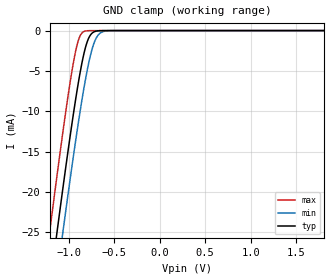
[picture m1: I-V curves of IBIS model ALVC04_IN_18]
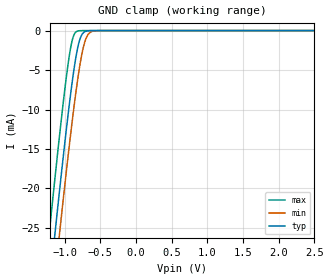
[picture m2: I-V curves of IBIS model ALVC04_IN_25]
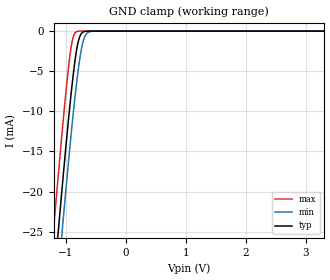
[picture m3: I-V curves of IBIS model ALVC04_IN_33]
| TEXAS INSTRUMENTS INCORPORATED
| Standard Linear and Logic Group
| IBIS Model of SN74ALVC04
| HEX INVERTER
| This file contains package information for the following:
|  SOIC 14-pin (D) package as [Component] ALVC04_D
|  TVSOP 14-pin (DGV) package as [Component] ALVC04_DGV
|  TSSOP 14-pin (PW) package as [Component] ALVC04_PW
| This device can be powered at the following Vccs:
|  1.8 volt Vcc
|  2.5 volt Vcc
|  3.3 volt Vcc
| This file provides unique models under the [Model Selector] for each Vcc.
| For operation at a specific Vcc, select the appropriate model after each
| [Model Selector] keyword.
[IBIS Ver]   3.2
[Comment char]  |_char
[File Name]   sn74alvc04.ibs
[File Rev]   1.1 | x_die
[Date]   March 8, 2002
[Source]   Data created from TI-SPICE simulations at TI-SLL.
[Notes]   The following is an IBIS list for the ALVC04.
   Please contact sllibis@ti.com with questions and
   comments concerning SLL IBIS models.
[Disclaimer] Property of Texas Instruments Incorporated.  Unauthorized
   reproduction and/or distribution is strictly prohibited.
   This product is protected under copyright law.
   Created  2002, (C) Copyright  2002, Texas Instruments
   Incorporated, All Rights Reserved
   UNLESS THERE IS A SIGNED, WRITTEN AGREEMENT TO THE
   CONTRARY, TEXAS INSTRUMENTS (TI) IS PROVIDING THE IBIS
   MODELS  AND WITHOUT ANY WARRANTY, EXPRESSED OR
   IMPLIED.  TI assumes no liability for:
   1) the accuracy of the IBIS models provided to your
   company;
   2) the proper functioning of these IBIS Models in your
   design or for any resulting applications; or
   3) infringement of patents, copyrights or intellectual
   property rights resulting from your use of these IBIS
   models.
   TI provides IBIS Models as a service to our customers.
   You and your company shall not distribute, sell or give
   these models to anyone else without prior written
   permission from TI.
   TI reserves the right to make changes to our products or
   to discontinue any semiconductor product or service
   without notice, and advises our customers to obtain the
   latest version of relevant information to verify, before
   placing orders, that the information being relied on is
   current.
   Please be aware that your receipt and use of the IBIS
   information provided shall serve as acceptance of these
   terms and conditions.  If you do not accept these terms,
   you should return or destroy the IBIS models and any
   other accompanying information immediately.
| Component ALVC04_D 14-pin SOIC
[Component]   ALVC04_D
[Manufacturer]   Texas Instruments, Inc.
[Package]
|   typ   min   max
R_pkg   3.100e-02   2.800e-02   3.400e-02
L_pkg   3.109e-09   2.462e-09   3.889e-09
C_pkg   4.730e-13   3.630e-13   6.280e-13
[Pin]   signal_name   model_name   R_pin   L_pin   C_pin
1   A1   ALVC04_IN   3.300e-02   3.854e-09   6.220e-13
2   Y1   ALVC04_OUT   3.200e-02   3.188e-09   4.730e-13
3   A2   ALVC04_IN   2.800e-02   2.462e-09   3.770e-13
4   Y2   ALVC04_OUT   3.100e-02   2.596e-09   3.630e-13
5   A3   ALVC04_IN   2.800e-02   2.521e-09   3.720e-13
6   Y3   ALVC04_OUT   3.400e-02   3.250e-09   4.760e-13
7   GND   GND   3.400e-02   3.889e-09   6.280e-13
8   Y4   ALVC04_OUT   3.400e-02   3.889e-09   6.280e-13
9   A4   ALVC04_IN   3.400e-02   3.250e-09   4.760e-13
10   Y5   ALVC04_OUT   2.800e-02   2.521e-09   3.720e-13
11   A5   ALVC04_IN   3.100e-02   2.596e-09   3.640e-13
12   Y6   ALVC04_OUT   2.800e-02   2.462e-09   3.770e-13
13   A6   ALVC04_IN   3.200e-02   3.188e-09   4.730e-13
14   VCC   POWER   3.300e-02   3.854e-09   6.220e-13
| Component ALVC04_DGV 14-pin TVSOP
[Component]   ALVC04_DGV
[Manufacturer]   Texas Instruments, Inc.
[Package]
|   typ   min   max
R_pkg   3.500e-02   2.000e-02   4.500e-02
L_pkg   2.499e-09   2.077e-09   2.966e-09
C_pkg   3.610e-13   3.050e-13   4.160e-13
[Pin]   signal_name   model_name   R_pin   L_pin   C_pin
1   A1   ALVC04_IN   2.700e-02   2.717e-09   3.730e-13
2   Y1   ALVC04_OUT   3.700e-02   2.434e-09   3.980e-13
3   A2   ALVC04_IN   3.400e-02   2.200e-09   3.160e-13
4   Y2   ALVC04_OUT   2.000e-02   2.077e-09   3.090e-13
5   A3   ALVC04_IN   3.000e-02   2.147e-09   3.050e-13
6   Y3   ALVC04_OUT   4.200e-02   2.580e-09   4.080e-13
7   GND   GND   3.900e-02   2.921e-09   3.850e-13
8   Y4   ALVC04_OUT   3.300e-02   2.841e-09   3.800e-13
9   A4   ALVC04_IN   4.200e-02   2.611e-09   4.100e-13
10   Y5   ALVC04_OUT   3.800e-02   2.331e-09   3.290e-13
11   A5   ALVC04_IN   2.600e-02   2.223e-09   3.190e-13
12   Y6   ALVC04_OUT   3.400e-02   2.259e-09   3.130e-13
13   A6   ALVC04_IN   4.500e-02   2.681e-09   4.160e-13
14   VCC   POWER   4.200e-02   2.966e-09   3.860e-13
| Component ALVC04_PW 14-pin TSSOP
[Component]   ALVC04_PW
[Manufacturer]   Texas Instruments, Inc.
[Package]
|   typ   min   max
R_pkg   3.200e-02   2.900e-02   3.500e-02
L_pkg   2.378e-09   2.170e-09   2.680e-09
C_pkg   3.140e-13   2.700e-13   3.350e-13
[Pin]   signal_name   model_name   R_pin   L_pin   C_pin
1   A1   ALVC04_IN   3.300e-02   2.618e-09   3.300e-13
2   Y1   ALVC04_OUT   3.100e-02   2.313e-09   3.170e-13
3   A2   ALVC04_IN   3.000e-02   2.310e-09   3.140e-13
4   Y2   ALVC04_OUT   3.100e-02   2.173e-09   2.720e-13
5   A3   ALVC04_IN   3.000e-02   2.204e-09   3.090e-13
6   Y3   ALVC04_OUT   3.200e-02   2.315e-09   3.170e-13
7   GND   GND   3.500e-02   2.680e-09   3.350e-13
8   Y4   ALVC04_OUT   3.300e-02   2.640e-09   3.330e-13
9   A4   ALVC04_IN   3.400e-02   2.347e-09   3.190e-13
10   Y5   ALVC04_OUT   2.900e-02   2.277e-09   3.130e-13
11   A5   ALVC04_IN   3.100e-02   2.170e-09   2.700e-13
12   Y6   ALVC04_OUT   3.100e-02   2.244e-09   3.110e-13
13   A6   ALVC04_IN   3.300e-02   2.343e-09   3.210e-13
14   VCC   POWER   3.500e-02   2.657e-09   3.320e-13
| Model ALVC04_IN
[Model Selector]   ALVC04_IN
ALVC04_IN_18   1.8 volt Vcc
ALVC04_IN_25   2.5 volt Vcc
ALVC04_IN_33   3.3 volt Vcc
| Model ALVC04_OUT
[Model Selector]   ALVC04_OUT
ALVC04_OUT_18   1.8 volt Vcc
ALVC04_OUT_25   2.5 volt Vcc
ALVC04_OUT_33   3.3 volt Vcc
| Models and submodels in the file (6): ALVC04_IN_18 (Input), ALVC04_IN_25 (Input), ALVC04_IN_33 (Input), ALVC04_OUT_18 (Output), ALVC04_OUT_25 (Output), ALVC04_OUT_33 (Output)
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[Model]   ALVC04_IN_18
Model_type  Input
Vinl=0.5775
Vinh=1.2675
| variable   typ   min   max
C_comp   3.07pF   2.60pF   3.69pF
[Temperature Range]   40   100   -40
| Ambient temperature   25   85   -40
[Voltage range]   1.8   1.65   1.95
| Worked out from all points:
|   GND clamp passes 1 mA (typ) near -0.78 V on its own axis
[GND Clamp]
| ALVC04_IN_18
|   Voltage   I(typ)   I(min)   I(max)
-1.8V     -85.6mA    -90.87mA   -78.93mA
-1.205V   -31.84mA   -37.3mA    -24.82mA
-1.125V   -24.91mA   -30.38mA   -17.89mA
-1.06V    -19.42mA   -24.86mA   -12.46mA
-980mV    -12.93mA   -18.26mA   -6.256mA
-925mV    -8.768mA   -13.92mA   -2.718mA
-880mV    -5.677mA   -10.55mA   -833.1uA
-835mV    -3.071mA   -7.417mA   -141.2uA
-780mV    -970.8uA   -4.107mA   -11.31uA
-725mV    -188.6uA   -1.712mA   -853.8nA
-615mV    -4.273uA   -110.7uA   -4.819nA
1.8V      3.325pA    5.318pA    3.026pA
[Model]   ALVC04_IN_25
Model_type  Input
Vinl=0.7
Vinh=1.7
| variable   typ   min   max
C_comp   3.07pF   2.36pF   3.76pF
[Temperature Range]   40   100   -40
| Ambient temperature   25   85   -40
[Voltage range]   2.5   2.3   2.7
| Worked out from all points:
|   GND clamp passes 1 mA (typ) near -0.78 V on its own axis
[GND Clamp]
| ALVC04_IN_25
|   Voltage   I(typ)   I(min)   I(max)
-2.5V     -150.5mA   -155.5mA   -144.1mA
-1.23V    -34.03mA   -39.49mA   -27.02mA
-1.2V     -31.4mA    -36.87mA   -24.38mA
-1.13V    -25.34mA   -30.81mA   -18.32mA
-1.07V    -20.26mA   -25.7mA    -13.28mA
-925mV    -8.768mA   -13.92mA   -2.718mA
-880mV    -5.677mA   -10.55mA   -833.1uA
-830mV    -2.824mA   -7.089mA   -113.2uA
-780mV    -970.8uA   -4.107mA   -11.31uA
-720mV    -160uA     -1.553mA   -674.8nA
-600mV    -2.528uA   -72.05uA   -2.381nA
2.5V      4.712pA    6.752pA    4.389pA
[Model]   ALVC04_IN_33
Model_type  Input
Vinl=0.8
Vinh=2.0
| variable   typ   min   max
C_comp   3.07pF   2.21pF   3.73pF
[Temperature Range]   40   100   -40
| Ambient temperature   25   85   -40
[Voltage range]   3.3   3   3.6
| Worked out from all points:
|   GND clamp passes 1 mA (typ) near -0.78 V on its own axis
[GND Clamp]
| ALVC04_IN_33
|   Voltage   I(typ)   I(min)   I(max)
-3.3V     -225.3mA   -230.1mA   -219.2mA
-1.215V   -32.71mA   -38.18mA   -25.7mA
-1.185V   -30.09mA   -35.56mA   -23.07mA
-1.125V   -24.91mA   -30.38mA   -17.89mA
-1.065V   -19.84mA   -25.28mA   -12.87mA
-920mV    -8.408mA   -13.54mA   -2.452mA
-875mV    -5.359mA   -10.19mA   -702.5uA
-825mV    -2.587mA   -6.765mA   -90.45uA
-775mV    -851.5uA   -3.845mA   -8.949uA
-715mV    -135.5uA   -1.404mA   -533.3nA
-585mV    -1.495uA   -46.71uA   -1.178nA
3.3V      6.303pA    8.434pA    5.93pA
